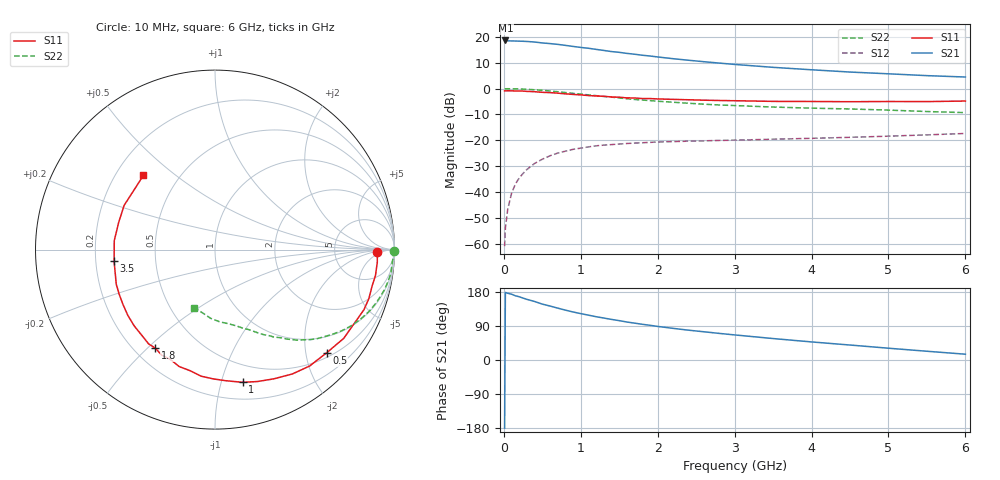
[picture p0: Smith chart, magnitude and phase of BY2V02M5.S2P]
! SIEMENS Small Signal Semiconductors
! BFY420
! Si NPN RF SIEGET Grounded Emitter Transistor in MICRO-X
! VCE = 2 V  IC = 2.5 mA
! Common Emitter S-Parameters:  October  1996
# GHz  S  MA  R  50
!  f  S11  S21  S12  S22
! GHz  MAG  ANG  MAG  ANG  MAG  ANG  MAG  ANG
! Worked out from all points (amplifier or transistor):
!   36 points, 10 MHz to 6 GHz, reference 50 ohm
!   highest |S21| = 18.6 dB at 20 MHz (marker M1)
!   |S21| within 3 dB of that: start of sweep to 1.095 GHz
!   unconditionally stable (mu >= 1): 3.812 GHz to end of sweep
!   at 250 MHz: K = 0.06, MSG = 25.5 dB, |S12| = -32.8 dB
!   at 1.4 GHz: K = 0.35, MSG = 18.0 dB, |S12| = -21.6 dB
!   at 6 GHz: K = 1.22, MAG = 8.1 dB, |S12| = -17.3 dB
!   S11 on the Smith chart (normalised r, x): 10 MHz: 20, -3; 500 MHz: 0.60, -2.43; 1 GHz: 0.34, -1.17; 1.8 GHz: 0.28, -0.53; 3.5 GHz: 0.28, -0.05; 6 GHz: 0.31, +0.39
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0.01  0.9052 -0.9  8.499 -179.7  0.0009 84.5  0.996 -0.5
0.02  0.905 -1.9  8.518 178.3  0.002 98.9  0.9903 -0.8
0.05  0.907 -4.4  8.372 176.1  0.0046 91.9  0.994 -2.3
0.1  0.9057 -9.1  8.338 173.7  0.0094 87.5  0.9894 -4.6
0.15  0.8984 -13.3  8.307 169.4  0.0143 82.1  0.9888 -6.9
0.2  0.8997 -17.6  8.261 166.9  0.0187 80.6  0.9845 -9.0
0.3  0.8831 -25.8  8.147 160.0  0.0273 75.2  0.9695 -13.5
0.4  0.8711 -34.6  7.939 154.4  0.0358 70.3  0.9486 -17.8
0.5  0.8471 -42.7  7.631 147.5  0.0431 66.6  0.9252 -21.8
0.7  0.8161 -58.1  7.16 136.9  0.0566 58.3  0.8698 -29.2
0.8  0.7913 -65.5  6.846 131.6  0.0617 54.0  0.8391 -32.6
1  0.7553 -78.2  6.249 122.4  0.0707 47.9  0.782 -38.2
1.1  0.7335 -85.1  6.018 118.3  0.0746 45.0  0.7557 -41.0
1.4  0.6889 -101.6  5.192 107.1  0.0827 38.2  0.6836 -47.6
1.6  0.6611 -112.0  4.79 100.2  0.0869 34.4  0.6372 -51.4
1.8  0.6422 -121.1  4.413 94.2  0.0897 31.5  0.6009 -54.5
2.2  0.6192 -136.6  3.783 83.5  0.0945 26.8  0.5454 -60.3
2.8  0.5887 -155.2  3.112 70.2  0.0995 22.6  0.482 -67.4
3.5  0.5659 -173.4  2.575 56.6  0.1051 19.8  0.4397 -74.7
4.5  0.5576 164.3  2.088 39.5  0.1143 17.1  0.4037 -86.1
5.5  0.5605 143.1  1.78 23.1  0.1275 14.8  0.3602 -100.8
6  0.5746 134.0  1.673 15.3  0.1357 13.2  0.3431 -109.5
